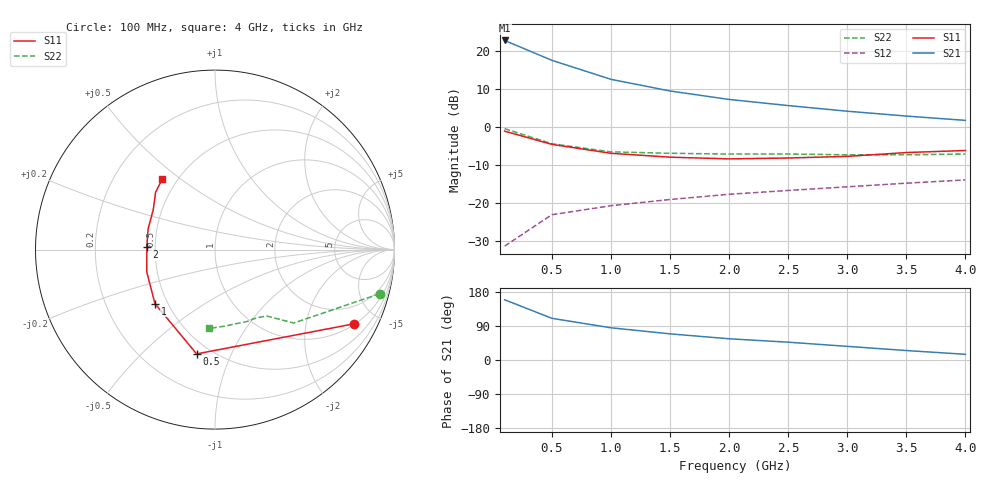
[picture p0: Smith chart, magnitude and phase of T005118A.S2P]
!AT-00511
!S-PARAMETERS at Vce=8V  Ic=5mA.  LAST UPDATED 07-21-92
!OBSOLETED Feb 1994 - nearest replacement: AT-41511
# ghz s ma r 50
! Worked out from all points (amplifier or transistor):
!   9 points, 100 MHz to 4 GHz, reference 50 ohm
!   highest |S21| = 22.8 dB at 100 MHz (marker M1)
!   |S21| within 3 dB of that: start of sweep to 329.5 MHz
!   unconditionally stable (mu >= 1): 1.438 GHz to end of sweep
!   at 500 MHz: K = 0.50, MSG = 20.3 dB, |S12| = -23.1 dB
!   at 2 GHz: K = 1.15, MAG = 10.2 dB, |S12| = -17.7 dB
!   at 4 GHz: K = 1.17, MAG = 5.3 dB, |S12| = -13.9 dB
!   lowest NFmin = 1.30 dB at 100 MHz
!   S11 on the Smith chart (normalised r, x): 100 MHz: 1.02, -3.75; 500 MHz: 0.42, -0.75; 1 GHz: 0.43, -0.32; 2 GHz: 0.45, +0.01; 4 GHz: 0.42, +0.43
0.1  0.88 -28.0  13.73 159.0  0.027 79.0  0.95 -15.0
0.5  0.59 -100.0  7.52 110.0  0.07 43.0  0.6 -43.0
1  0.45 -138.0  4.23 85.0  0.092 41.0  0.47 -52.0
1.5  0.4 -162.0  2.97 69.0  0.111 42.0  0.45 -57.0
2  0.38 178.0  2.3 56.0  0.13 41.0  0.44 -62.0
2.5  0.39 163.0  1.91 47.0  0.146 44.0  0.44 -65.0
3  0.41 147.0  1.61 36.0  0.163 44.0  0.43 -73.0
3.5  0.46 136.0  1.39 25.0  0.182 39.0  0.43 -83.0
4  0.49 127.0  1.22 15.0  0.201 37.0  0.44 -94.0
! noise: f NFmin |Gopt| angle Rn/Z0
0.1  1.3  0.5  4  0.45
0.5  1.4  0.46  19  0.44
1  1.8  0.37  38  0.42
2  2.7  0.22  87  0.37
4  4.4  0.2  -154  0.42
